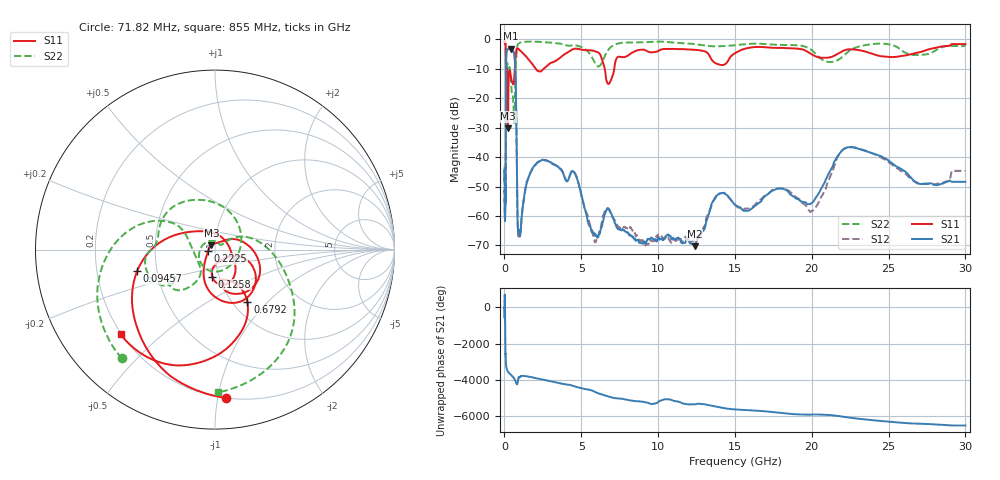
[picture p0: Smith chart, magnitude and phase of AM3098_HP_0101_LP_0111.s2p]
! Date/Time: Thu, Feb 28, 2019 8:36 AM
! Network Analyzer: Agilent Technologies E8364B Rev: A.07.50.67
! Sweep from 0.010 to 30.000 GHz, 1601 Points, Sweep Type: LOG
! Power Supply: 5.022 V, 0.001 A
# Hz S DB R 50
!freq MagS11 AngS11 MagS21 AngS21 MagS12 AngS12 MagS22 AngS22
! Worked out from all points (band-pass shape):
!   1601 points, 10 MHz to 30 GHz, reference 50 ohm
!   highest |S21| = -3.10 dB at 413.9 MHz (marker M1); lowest = -70.2 dB at 12.37 GHz (marker M2)
!   |S21| within 3 dB of the highest: 113.6 MHz to 660.3 MHz (546.8 MHz wide, 141 % of centre)
!   lowest |S11| = -30.2 dB at 229.3 MHz (marker M3), VSWR 1.06, Z = 48 + j2.21 ohm
!   |S11| at or under -10 dB: 176.5 MHz to 671.4 MHz (494.9 MHz wide, 117 % of centre); 2.04 GHz to 2.549 GHz (509.5 MHz wide, 22.2 % of centre); 6.527 GHz to 7.145 GHz (618.9 MHz wide, 9.05 % of centre)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
!   |S22| runs from -28.3 to -0.5 dB; largest |S21 - S12| = 0.011
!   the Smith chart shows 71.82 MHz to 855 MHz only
!   S11 on the Smith chart (normalised r, x): 71.82 MHz: 0.20, -1.05; 94.57 MHz: 0.39, -0.11; 125.8 MHz: 0.93, -0.29; 222.5 MHz: 0.92, -0.01; 679.2 MHz: 1.16, -0.77; 855 MHz: 0.20, -0.37
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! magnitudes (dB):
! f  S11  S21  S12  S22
! 10 MHz  -0.4  -47.9  -43.2  -0.5
! 38.04 MHz  -0.5  -59.9  -59.8  -0.9
! 71.82 MHz  -1.6  -54.4  -52.2  -2.0
! 82.62 MHz  -2.7  -48.6  -49.8  -2.9
! 94.57 MHz  -7.0  -23.5  -23.5  -7.9
! 125.8 MHz  -16.4  -4.8  -4.8  -10.1
! 144.7 MHz  -16.4  -3.9  -3.8  -10.9
! 183.1 MHz  -10.6  -3.7  -3.6  -8.0
! 222.5 MHz  -28.0  -3.3  -3.2  -9.3
! 229.3 MHz  -30.2  -3.2  -3.2  -9.5
! 413.9 MHz  -12.4  -3.1  -3.1  -13.0
! 550.5 MHz  -15.2  -3.8  -3.7  -19.3
! 679.2 MHz  -9.3  -7.2  -7.2  -21.6
! 747 MHz  -4.8  -18.0  -17.9  -8.0
! 855 MHz  -3.0  -61.6  -61.8  -2.0
! 2.084 GHz  -10.3  -42.3  -42.1  -0.8
! 7.926 GHz  -5.8  -65.5  -64.0  -1.1
! 12.37 GHz  -3.5  -70.2  -68.0  -1.6
! 14.02 GHz  -8.6  -52.3  -52.4  -2.3
! 20.1 GHz  -5.4  -55.1  -58.0  -4.1
! 22.56 GHz  -3.4  -36.6  -36.6  -3.5
! 30 GHz  -1.6  -48.4  -44.6  -2.3
